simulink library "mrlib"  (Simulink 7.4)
settings: Solver=ode45  SolverMode=SingleTasking  StartTime=0.0  StopTime=10.0  RelTol=1e-3
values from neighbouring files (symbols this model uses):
  D = str2num(get(h,'string'))    [acttrcalc1.m]
  fr0 = [phidr phiqr]    [imdef0vec.m]    (also in imdef1vec.m; imdefrotflux.m = sqrt(phidr^2+phiqr^2); imdefSIvec1.m)
  fs0 = fs    [calc0.m]    (also in imdef0vec.m = [phids phiqs]; imdef1vec.m = [phids phiqs]; imdefrotflux.m = [fs0d fs0q]; imdefSIvec1.m = [phids phiqs])
  gam = 2*pi/3    (= 2.09439510239)    [IMabc2.m]    (also in IMabcf0.m; IMabcf1.m; imabcparam.m; IMabcrun0.m)
  ic = [fs0 fr0]    [imdef0vec.m]    (also in imdef1vec.m; imdef2vec.m = F; imic2.m = [phids phiqs phidr phiqr n0]'; imic3.m = [phids phiqs phidr phiqr n0]')
  Lm1 = 2/3*Lm    [IMabcf0.m]    (also in IMabcf1.m; imabcparam.m = 0.0564666666667; IMabcrun0.m = 0.0564666666667; IMabcrun1.m = 0.0564666666667)
  Lr = Lrl+Lm    (= 4.6)    [IMabc2.m]    (also in IMabcf0.m = Lrl+Lm1; IMabcf1.m = Lrl+Lm1; imabcparam.m = 0.0589666666667; IMcur0.m)
  Lrr = [Lr   -Lm/2 -Lm/2    [IMabc2.m]    (also in IMabcf0.m = [Lr   -Lm1/2 -Lm1/2; IMabcf1.m = [Lr   -Lm1/2 -Lm1/2)
  Ls = Lsl+Lm    (= 4.6)    [IMabc2.m]    (also in IMabcf0.m = Lsl+Lm1; IMabcf1.m = Lsl+Lm1; imabcparam.m = 0.0589666666667; IMcur0.m)
  Lss = [Ls   -Lm/2 -Lm/2    [IMabc2.m]    (also in IMabcf0.m = [Ls   -Lm1/2 -Lm1/2; IMabcf1.m = [Ls   -Lm1/2 -Lm1/2)
  p = cos(beta-alpha)    [abcRwdg.m]    (also in alternator.m = 0:pi/20:2*pi; altwdgs.m = 0:pi/20:2*pi; brushlessdcB.m = 0:pi/100:2*pi; brushlessdcnew.m = 0:pi/100:2*pi)
  R = str2num(get(h,'string'))    [acttrcalc1.m]    (also in IMabc2.m = diag([Rs Rs Rs Rr Rr Rr]); IMabcf0.m = diag([Rs Rs Rs Rr Rr Rr]); IMabcf1.m = diag([Rs Rs Rs Rr Rr Rr]); IMcurf0.m = diag([Rs Rs Rr Rr]))
  Ra = .95    (= 0.95)    [altwdgs.m]    (also in Ccurverun.m = 0.018)
  Rr = input('Rotor resistance)[default = 2] =')    [Actac.m]    (also in im1phase.m = 0.3; im3d.m = eval(get(hRr,'String')); IMabc2.m = 0.02; imabcparam.m = 0.408)
  Rs = eval(get(hRs,'String'))    [im3d.m]    (also in IMabc2.m = 0.01; imabcparam.m = 0.531; IMabcrun0.m = 0.531; IMabcrun1.m = 0.531)
  Vm = Vll*sqrt(2/3)    [imabcparam.m]
  wo = 2*pi*freq0    [calc0.m]    (also in IMabc2.m = 376.991118431; imabcparam.m = 376.991118431; IMabcrun0.m = 376.991118431; IMabcrun1.m = 376.991118431)
undefined symbols (not defined in the file or in its folder): fa0, fk0, ifo, L_1, Laf, Lakd, Lakq, phif0, Rf, Rkd, Rkq, Row, vector
libraries: simulink x4

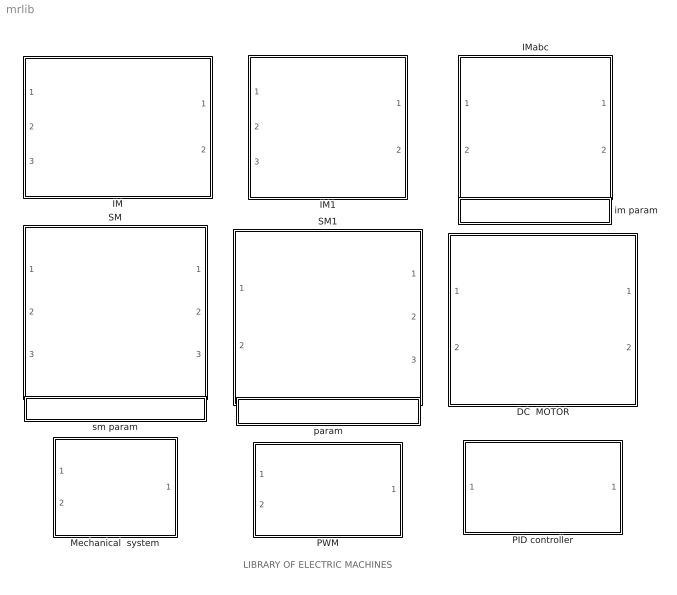
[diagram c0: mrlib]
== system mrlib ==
  note: LIBRARY OF ELECTRIC MACHINES
  DC  MOTOR : Subsystem  mask{Ra=2.0, La=5.2e-3, J=1.5e-4, Bm=1e-3, K=0.1}
      mask prompts: Ra "Armature resistance [ohm]"; La "Armature inductance [H]"; J "Moment of inertia [Kg.m^2]"; Bm "Frictional torque cefficient"; K "Electromechanical coupling coefficient [N.m/A]"
  IM : Subsystem  mask{Rs=0.02, Rr=0.01, Lsl=0.1, Lrl=0.1, Lm=5, wo=2*pi*60}
      mask prompts: Rs "Stator resistance [pu]"; Rr "Rotor resistance [pu]"; Lsl "Stator leakage inductance [pu]"; Lrl "Rotor leakage inductance [pu]"; Lm "Magnetizing inductance [pu]"; wo "Base frequency [rad/s]"
      mask help: Induction motor state space model in arbitrary reference frame. Parameters are expressed in per unit.
  IM1 : Subsystem  mask{Rs=0.5, Rr=0.5, Lsl=3e-3, Lrl=3e-3, Lm=100e-3, p=4, wo=2*pi*60}
      mask prompts: Rs "Stator resistance [Ohm]"; Rr "Rotor resistance [Ohm]"; Lsl "Stator leakage inductance [H]"; Lrl "Rotor leakage inductance [H]"; Lm "Magnetizing inductance [H]"; p "Number of poles"; wo "Base frequency [rad/s]"
  IMabc : Subsystem
  Mechanical  system : Subsystem  mask{H=0.3, B1=1e-5, B2=0, a=2}
      mask prompts: H "Inertia constant [s]"; B1 "Viscous damping coefficient"; B2 "Fan load factor"; a "Fan load exponent"
  PID controller : Subsystem  mask{Kp=1, Ki=10, Kd=0.1, sat=inf}
      mask prompts: Kp "Proportional gain (Kp)"; Ki "Integral gain (Ki)"; Kd "Derivative gain (Kd)"; sat "Saturation limit [pu]"
      mask help: Proportional-Integral Speed Controller
  PWM : Subsystem
  SM : Subsystem
  SM1 : Subsystem
  im param : Subsystem
  param : Subsystem
  sm param : Subsystem

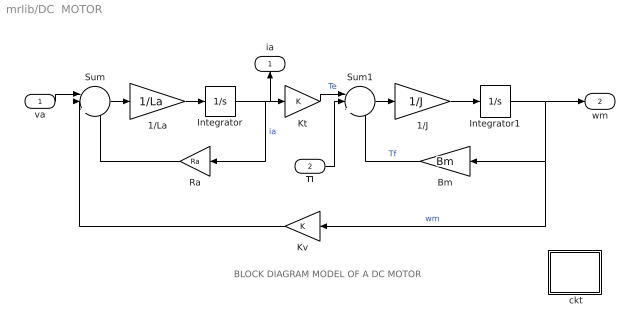
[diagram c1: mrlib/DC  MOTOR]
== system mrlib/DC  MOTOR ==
  note: BLOCK DIAGRAM MODEL OF A DC MOTOR
  va : Inport  OutDataType=sfix(16)  OutScaling=2^0
  Tl : Inport  Port=2  OutDataType=sfix(16)  OutScaling=2^0
  " ckt" : Subsystem
  1/J : Gain  Gain=1/J  ParameterDataType=sfix(16)  ParameterScaling=2^0  OutDataType=sfix(16)  OutScaling=2^0
  1/La : Gain  Gain=1/La  ParameterDataType=sfix(16)  ParameterScaling=2^0  OutDataType=sfix(16)  OutScaling=2^0
  Bm : Gain  Gain=Bm  ParameterDataType=sfix(16)  ParameterScaling=2^0  OutDataType=sfix(16)  OutScaling=2^0
  Integrator : Integrator
  Integrator1 : Integrator
  Kt : Gain  Gain=K  ParameterDataType=sfix(16)  ParameterScaling=2^0  OutDataType=sfix(16)  OutScaling=2^0
  Kv : Gain  Gain=K  ParameterDataType=sfix(16)  ParameterScaling=2^0  OutDataType=sfix(16)  OutScaling=2^0
  Ra : Gain  Gain=Ra  ParameterDataType=sfix(16)  ParameterScaling=2^0  OutDataType=sfix(16)  OutScaling=2^0
  Sum : Sum  Inputs=||+--  OutDataType=sfix(16)  OutScaling=2^0
  Sum1 : Sum  Inputs=||+--  OutDataType=sfix(16)  OutScaling=2^0
  ia : Outport
  wm : Outport  Port=2
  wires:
  Kv/1 -> Sum/2
  Ra/1 -> Sum/3
  Kt/1 -> Sum1/1  "Te"
  Bm/1 -> Sum1/3  "Tf"
  Sum/1 -> 1/La/1
  1/La/1 -> Integrator/1
  Integrator/1 -> Ra/1, Kt/1, ia/1  "ia"
  Sum1/1 -> 1/J/1
  1/J/1 -> Integrator1/1
  va/1 -> Sum/1
  Tl/1 -> Sum1/2
  Integrator1/1 -> Bm/1, Kv/1, wm/1  "wm"

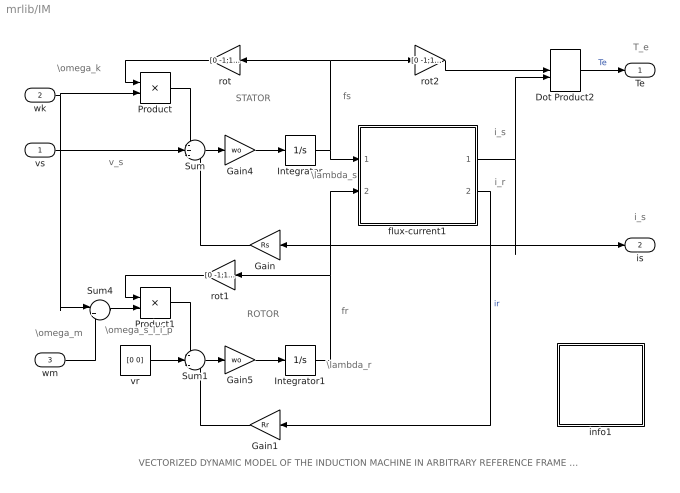
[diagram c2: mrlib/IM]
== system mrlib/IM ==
  note: VECTORIZED DYNAMIC MODEL OF THE INDUCTION MACHINE IN ARBITRARY REFERENCE FRAME (per unit formulation)
  note: fr
  note: fs
  note: STATOR
  note: ROTOR
  note: \omega_s_l_i_p
  note: T_e
  note: i_s
  note: i_s
  note: i_r
  note: \omega_m
  note: \lambda_s
  note: \lambda_r
  note: v_s
  note: \omega_k
  vs : Inport  OutDataType=sfix(16)  OutScaling=2^0
  wk : Inport  Port=2  OutDataType=sfix(16)  OutScaling=2^0
  wm : Inport  Port=3  OutDataType=sfix(16)  OutScaling=2^0
  Dot Product2 : DotProduct  OutDataType=fixdt(1, 16)  OutScaling=2^-10
  Gain : Gain  Gain=Rs  ParameterDataType=sfix(16)  ParameterScaling=2^0  OutDataType=sfix(16)  OutScaling=2^0
  Gain1 : Gain  Gain=Rr  ParameterDataType=sfix(16)  ParameterScaling=2^0  OutDataType=sfix(16)  OutScaling=2^0
  Gain4 : Gain  Gain=wo  ParameterDataType=sfix(16)  ParameterScaling=2^0  OutDataType=sfix(16)  OutScaling=2^0
  Gain5 : Gain  Gain=wo  ParameterDataType=sfix(16)  ParameterScaling=2^0  OutDataType=sfix(16)  OutScaling=2^0
  Integrator : Integrator  InitialCondition=[ic(1) ic(2)]
  Integrator1 : Integrator  InitialCondition=[ic(3) ic(4)]
  Product : Product  OutDataType=sfix(16)  OutScaling=2^0
  Product1 : Product  OutDataType=sfix(16)  OutScaling=2^0
  Sum : Sum  Inputs=-+-  OutDataType=sfix(16)  OutScaling=2^0
  Sum1 : Sum  Inputs=-+-  OutDataType=sfix(16)  OutScaling=2^0
  Sum4 : Sum  Inputs=|+-  OutDataType=sfix(16)  OutScaling=2^0
  flux-current1 : Subsystem
  info1 : Subsystem
  rot : Gain  Gain=[0 -1;1 0]  Multiplication=Matrix(K*u)  ParameterDataType=sfix(16)  ParameterScaling=2^0  OutDataType=sfix(16)  OutScaling=2^0
  rot1 : Gain  Gain=[0 -1;1 0]  Multiplication=Matrix(K*u)  ParameterDataType=sfix(16)  ParameterScaling=2^0  OutDataType=sfix(16)  OutScaling=2^0
  rot2 : Gain  Gain=[0 -1;1 0]  Multiplication=Matrix(K*u)  ParameterDataType=sfix(16)  ParameterScaling=2^0  OutDataType=sfix(16)  OutScaling=2^0
  vr : Constant  Value=[0 0]  OutDataType=sfix(16)  OutScaling=2^0
  Te : Outport
  is : Outport  Port=2
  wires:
  wm/1 -> Sum4/2
  wk/1 -> Sum4/1, Product/2
  vs/1 -> Sum/2
  Dot Product2/1 -> Te/1  "Te"
  flux-current1/1(is) -> Dot Product2/2, is/1, Gain/1
  Gain5/1 -> Integrator1/1
  Sum1/1 -> Gain5/1
  Gain4/1 -> Integrator/1
  Sum/1 -> Gain4/1
  Sum4/1 -> Product1/2
  rot2/1 -> Dot Product2/1
  rot/1 -> Product/1
  Product/1 -> Sum/1
  rot1/1 -> Product1/1
  Product1/1 -> Sum1/1
  Integrator1/1 -> flux-current1/2(fr), rot1/1
  Integrator/1 -> rot2/1, rot/1, flux-current1/1(fs)
  flux-current1/2(ir) -> Gain1/1  "ir"
  Gain1/1 -> Sum1/3
  vr/1 -> Sum1/2
  Gain/1 -> Sum/3

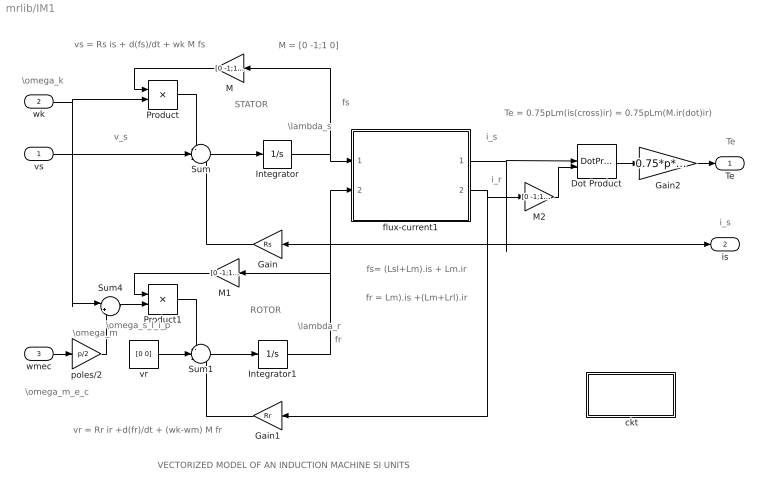
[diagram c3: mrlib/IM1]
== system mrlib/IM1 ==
  note: ROTOR
  note: STATOR
  note: fs
  note: VECTORIZED MODEL OF AN INDUCTION MACHINE SI UNITS
  note: vs = Rs is + d(fs)/dt + wk M fs
  note: vr = Rr ir +d(fr)/dt + (wk-wm) M fr
  note: fs= (Lsl+Lm).is + Lm.ir
  note: fr = Lm).is +(Lm+Lrl).ir
  note: Te = 0.75pLm(is(cross)ir) = 0.75pLm(M.ir(dot)ir)
  note: M = [0 -1;1 0]
  note: fr
  note: Te
  note: \lambda_s
  note: \lambda_r
  note: i_s
  note: i_s
  note: i_r
  note: \omega_m
  note: \omega_m_e_c
  note: \omega_k
  note: v_s
  note: \omega_s_l_i_p
  vs : Inport  OutDataType=sfix(16)  OutScaling=2^0
  wk : Inport  Port=2  OutDataType=sfix(16)  OutScaling=2^0
  wmec : Inport  Port=3  OutDataType=sfix(16)  OutScaling=2^0
  " ckt" : Subsystem
  Dot Product : DotProduct  OutDataType=fixdt(1, 16)  OutScaling=2^-10
  Gain : Gain  Gain=Rs  ParameterDataType=sfix(16)  ParameterScaling=2^0  OutDataType=sfix(16)  OutScaling=2^0
  Gain1 : Gain  Gain=Rr  ParameterDataType=sfix(16)  ParameterScaling=2^0  OutDataType=sfix(16)  OutScaling=2^0
  Gain2 : Gain  Gain=0.75*p*Lm  ParameterDataType=sfix(16)  ParameterScaling=2^0  OutDataType=sfix(16)  OutScaling=2^0
  Integrator : Integrator  InitialCondition=fs0
  Integrator1 : Integrator  InitialCondition=fr0
  M : Gain  Gain=[0 -1;1 0]  Multiplication=Matrix(K*u)  ParameterDataType=sfix(16)  ParameterScaling=2^0  OutDataType=sfix(16)  OutScaling=2^0
  M1 : Gain  Gain=[0 -1;1 0]  Multiplication=Matrix(K*u)  ParameterDataType=sfix(16)  ParameterScaling=2^0  OutDataType=sfix(16)  OutScaling=2^0
  M2 : Gain  Gain=[0 -1;1 0]  Multiplication=Matrix(K*u)  ParameterDataType=sfix(16)  ParameterScaling=2^0  OutDataType=sfix(16)  OutScaling=2^0
  Product : Product  OutDataType=sfix(16)  OutScaling=2^0
  Product1 : Product  OutDataType=sfix(16)  OutScaling=2^0
  Sum : Sum  Inputs=-+-  OutDataType=sfix(16)  OutScaling=2^0
  Sum1 : Sum  Inputs=-+-  OutDataType=sfix(16)  OutScaling=2^0
  Sum4 : Sum  Inputs=|+-  OutDataType=sfix(16)  OutScaling=2^0
  flux-current1 : Subsystem
  poles/2 : Gain  Gain=p/2  ParameterDataType=sfix(16)  ParameterScaling=2^0  OutDataType=sfix(16)  OutScaling=2^0
  vr : Constant  Value=[0 0]  OutDataType=sfix(16)  OutScaling=2^0
  Te : Outport
  is : Outport  Port=2
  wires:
  Gain/1 -> Sum/3
  vr/1 -> Sum1/2
  Gain1/1 -> Sum1/3
  Integrator/1 -> M/1, flux-current1/1(fs)
  Integrator1/1 -> flux-current1/2(fr), M1/1
  Product1/1 -> Sum1/1
  M1/1 -> Product1/1
  Product/1 -> Sum/1
  M/1 -> Product/1
  Sum4/1 -> Product1/2
  vs/1 -> Sum/2
  wk/1 -> Product/2, Sum4/1
  Sum1/1 -> Integrator1/1
  Sum/1 -> Integrator/1
  flux-current1/1(is) -> Gain/1, is/1, Dot Product/1
  Dot Product/1 -> Gain2/1
  Gain2/1 -> Te/1
  wmec/1 -> poles/2/1
  poles/2/1 -> Sum4/2
  M2/1 -> Dot Product/2
  flux-current1/2(ir) -> M2/1, Gain1/1

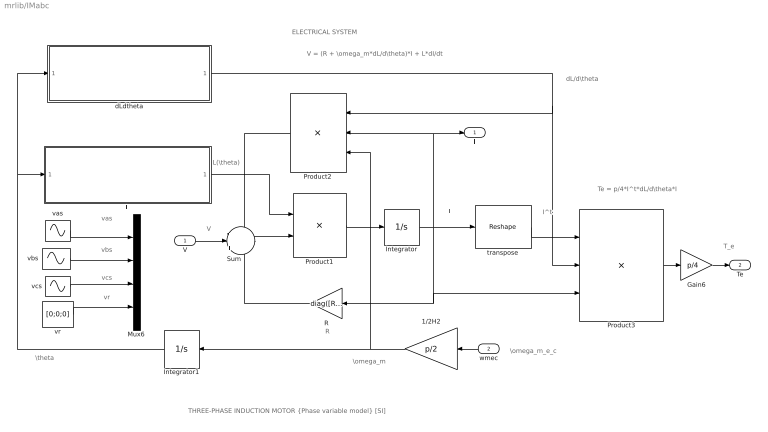
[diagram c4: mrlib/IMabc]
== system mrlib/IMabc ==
  note: I
  note: I^t
  note: ELECTRICAL SYSTEM
  note: V
  note: \omega_m
  note: \theta
  note: T_e
  note: dL/d\theta
  note: R
  note: V = (R + \omega_m*dL/d\theta)*I + L*dI/dt
  note: Te = p/4*I^t*dL/d\theta*I
  note: L(\theta)
  note: \omega_m_e_c
  note: THREE-PHASE INDUCTION MOTOR {Phase variable model} [SI]
  note: vas
  note: vbs
  note: vcs
  note: vr
  V : Inport  OutDataType=sfix(16)  OutScaling=2^0
  wmec : Inport  Port=2  OutDataType=sfix(16)  OutScaling=2^0
  1/2H2 : Gain  Gain=p/2  ParameterDataType=sfix(16)  ParameterScaling=2^0  OutDataType=sfix(16)  OutScaling=2^0
  Gain6 : Gain  Gain=p/4  ParameterDataType=sfix(16)  ParameterScaling=2^0  OutDataType=sfix(16)  OutScaling=2^0
  Integrator : Integrator  InitialCondition=[0 ;0 ;0; 0 ;0 ;0]
  Integrator1 : Integrator
  L : Subsystem
  Mux6 : Mux
  Product1 : Product  Inputs=/*  Multiplication=Matrix(*)  OutDataType=sfix(16)  OutScaling=2^0
  Product2 : Product  Inputs=***  Multiplication=Matrix(*)  OutDataType=sfix(16)  OutScaling=2^0
  Product3 : Product  Inputs=3  Multiplication=Matrix(*)  OutDataType=sfix(16)  OutScaling=2^0
  R : Gain  Gain=diag([Rs Rs Rs Rr Rr Rr])  Multiplication=Matrix(K*u)  ParameterDataType=sfix(16)  ParameterScaling=2^0  OutDataType=sfix(16)  OutScaling=2^0
  Sum : Sum  Inputs=-|+|-  OutDataType=sfix(16)  OutScaling=2^0
  dLdtheta : Subsystem
  transpose : Reshape  OutputDimensionality=Row vector (2-D)  OutputDimensions=[1,6]
  vas : Sin  Amplitude=Vm  Bias=0  Frequency=wo  Phase=pi/2  Samples=10  SampleTime=0
  vbs : Sin  Amplitude=Vm  Bias=0  Frequency=wo  Phase=pi/2-gam  Samples=10  SampleTime=0
  vcs : Sin  Amplitude=Vm  Bias=0  Frequency=wo  Phase=pi/2+gam  Samples=10  SampleTime=0
  vr : Constant  Value=[0;0;0]  VectorParams1D=off  OutDataType=sfix(16)  OutScaling=2^0
  I : Outport
  Te : Outport  Port=2
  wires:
  Product1/1 -> Integrator/1
  Integrator/1 -> Product3/3, R/1, transpose/1, Product2/2, I/1
  Sum/1 -> Product1/2
  R/1 -> Sum/3
  transpose/1 -> Product3/1
  Product2/1 -> Sum/1
  dLdtheta/1(dLdtheta) -> Product3/2, Product2/1
  Product3/1 -> Gain6/1
  1/2H2/1 -> Integrator1/1, Product2/3
  Integrator1/1 -> dLdtheta/1(theta1), L/1(theta)
  L/1(L) -> Product1/1
  V/1 -> Sum/2
  Gain6/1 -> Te/1
  wmec/1 -> 1/2H2/1
  vr/1 -> Mux6/4
  vcs/1 -> Mux6/3
  vbs/1 -> Mux6/2
  vas/1 -> Mux6/1
  Mux6/1 -> ?

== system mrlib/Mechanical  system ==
  note: fan-type load
  Tl : Inport  OutDataType=sfix(16)  OutScaling=2^0
  Te : Inport  Port=2  OutDataType=sfix(16)  OutScaling=2^0
  1/2H : Gain  Gain=1/(2*H)  ParameterDataType=sfix(16)  ParameterScaling=2^0  OutDataType=sfix(16)  OutScaling=2^0
  Bm : Gain  Gain=B1  ParameterDataType=sfix(16)  ParameterScaling=2^0  OutDataType=sfix(16)  OutScaling=2^0
  Integrator : Integrator  InitialCondition=.82
  Sum : Sum  Inputs=-+-  OutDataType=sfix(16)  OutScaling=2^0
  Sum1 : Sum  Inputs=|++  OutDataType=sfix(16)  OutScaling=2^0
  Tm : Fcn  Expr=B2*abs(u)^a
  wm : Outport
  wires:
  Tl/1 -> Sum/1
  Te/1 -> Sum/2
  Integrator/1 -> wm/1, Bm/1, Tm/1
  Sum/1 -> 1/2H/1
  1/2H/1 -> Integrator/1
  Bm/1 -> Sum1/1
  Sum1/1 -> Sum/3
  Tm/1 -> Sum1/2

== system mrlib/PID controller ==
  note: antiwindup by clamping integrator
  note: limiter
  error : Inport  OutDataType=sfix(16)  OutScaling=2^0
  Derivative : Derivative
  Gain : Gain  Gain=Ki  ParameterDataType=sfix(16)  ParameterScaling=2^0  OutDataType=sfix(16)  OutScaling=2^0
  Gain1 : Gain  Gain=Kp  ParameterDataType=sfix(16)  ParameterScaling=2^0  OutDataType=sfix(16)  OutScaling=2^0
  Gain2 : Gain  Gain=Kd  ParameterDataType=sfix(16)  ParameterScaling=2^0  OutDataType=sfix(16)  OutScaling=2^0
  Integrator : Integrator  LimitOutput=on  UpperSaturationLimit=sat  LowerSaturationLimit=-sat
  Saturation : Saturate  UpperLimit=sat  LowerLimit=-sat
  Sum : Sum  Inputs=+++  OutDataType=sfix(16)  OutScaling=2^0
  control : Outport  InitialOutput=0
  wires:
  Gain1/1 -> Sum/1
  Gain/1 -> Integrator/1
  error/1 -> Gain/1, Gain1/1, Gain2/1
  Sum/1 -> Saturation/1
  Saturation/1 -> control/1
  Integrator/1 -> Sum/2
  Gain2/1 -> Derivative/1
  Derivative/1 -> Sum/3

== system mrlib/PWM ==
  control : Inport  OutDataType=sfix(16)  OutScaling=2^0
  frequency : Inport  Port=2  OutDataType=sfix(16)  OutScaling=2^0
  Clock : Clock
  Mux : Mux  Inputs=2
  Sum2 : Sum  Inputs=|+-  OutDataType=sfix(16)  OutScaling=2^0
  saw : Fcn  Expr=1/pi*atan(tan((2*pi*u(1)*u(2)-pi)/2))+0.5
  step : Relay  OutDataType=sfix(16)  OutScaling=2^0
  Output : Outport
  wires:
  Clock/1 -> Mux/2
  Mux/1 -> saw/1
  control/1 -> Sum2/1
  frequency/1 -> Mux/1
  saw/1 -> Sum2/2
  step/1 -> Output/1
  Sum2/1 -> step/1

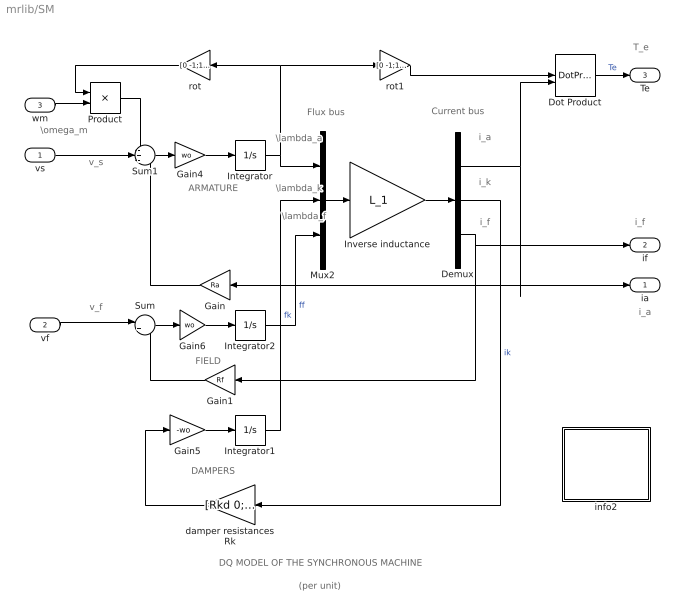
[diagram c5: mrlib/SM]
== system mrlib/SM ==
  note: DAMPERS
  note: ARMATURE
  note: i_f
  note: FIELD
  note: DQ MODEL OF THE SYNCHRONOUS MACHINE
  note: Flux bus
  note: Current bus
  note: (per unit)
  note: v_s
  note: T_e
  note: \lambda_a
  note: \lambda_k
  note: \lambda_f
  note: \omega_m
  note: v_f
  note: i_k
  note: i_a
  note: i_a
  note: i_f
  vs : Inport  OutDataType=sfix(16)  OutScaling=2^0
  vf : Inport  Port=2  OutDataType=sfix(16)  OutScaling=2^0
  wm : Inport  Port=3  OutDataType=sfix(16)  OutScaling=2^0
  Demux : Demux  Outputs=3
  Dot Product : DotProduct  OutDataType=fixdt(1, 16)  OutScaling=2^-10
  Gain : Gain  Gain=Ra  ParameterDataType=sfix(16)  ParameterScaling=2^0  OutDataType=sfix(16)  OutScaling=2^0
  Gain1 : Gain  Gain=Rf  ParameterDataType=sfix(16)  ParameterScaling=2^0  OutDataType=sfix(16)  OutScaling=2^0
  Gain4 : Gain  Gain=wo  ParameterDataType=sfix(16)  ParameterScaling=2^0  OutDataType=sfix(16)  OutScaling=2^0
  Gain5 : Gain  Gain=-wo  ParameterDataType=sfix(16)  ParameterScaling=2^0  OutDataType=sfix(16)  OutScaling=2^0
  Gain6 : Gain  Gain=wo  ParameterDataType=sfix(16)  ParameterScaling=2^0  OutDataType=sfix(16)  OutScaling=2^0
  Integrator : Integrator  InitialCondition=fa0
  Integrator1 : Integrator  InitialCondition=fk0
  Integrator2 : Integrator  InitialCondition=phif0
  Inverse inductance : Gain  Gain=L_1  Multiplication=Matrix(K*u)  ParameterDataType=sfix(16)  ParameterScaling=2^0  OutDataType=sfix(16)  OutScaling=2^0
  Mux2 : Mux  Inputs=3
  Product : Product  OutDataType=sfix(16)  OutScaling=2^0
  Sum : Sum  Inputs=|+-  OutDataType=sfix(16)  OutScaling=2^0
  Sum1 : Sum  Inputs=-+-  OutDataType=sfix(16)  OutScaling=2^0
  damper resistances Rk : Gain  Gain=[Rkd 0;0 Rkq]  Multiplication=Matrix(K*u)  ParameterDataType=sfix(16)  ParameterScaling=2^0  OutDataType=sfix(16)  OutScaling=2^0
  info2 : Subsystem
  rot : Gain  Gain=[0 -1;1 0]  Multiplication=Matrix(K*u)  ParameterDataType=sfix(16)  ParameterScaling=2^0  OutDataType=sfix(16)  OutScaling=2^0
  rot1 : Gain  Gain=[0 -1;1 0]  Multiplication=Matrix(K*u)  ParameterDataType=sfix(16)  ParameterScaling=2^0  OutDataType=sfix(16)  OutScaling=2^0
  ia : Outport
  if : Outport  Port=2
  Te : Outport  Port=3
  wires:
  Product/1 -> Sum1/1
  rot/1 -> Product/1
  Gain5/1 -> Integrator1/1
  damper resistances Rk/1 -> Gain5/1
  Integrator/1 -> Mux2/1, rot/1, rot1/1
  Sum1/1 -> Gain4/1
  Gain4/1 -> Integrator/1
  vs/1 -> Sum1/2
  Gain/1 -> Sum1/3
  Gain6/1 -> Integrator2/1
  Sum/1 -> Gain6/1
  vf/1 -> Sum/1
  Gain1/1 -> Sum/2
  rot1/1 -> Dot Product/1
  Demux/1 -> Gain/1, ia/1, Dot Product/2
  Dot Product/1 -> Te/1  "Te"
  Mux2/1 -> Inverse inductance/1
  Inverse inductance/1 -> Demux/1
  Integrator1/1 -> Mux2/2  "fk"
  Integrator2/1 -> Mux2/3  "ff"
  Demux/2 -> damper resistances Rk/1  "ik"
  Demux/3 -> if/1, Gain1/1
  wm/1 -> Product/2

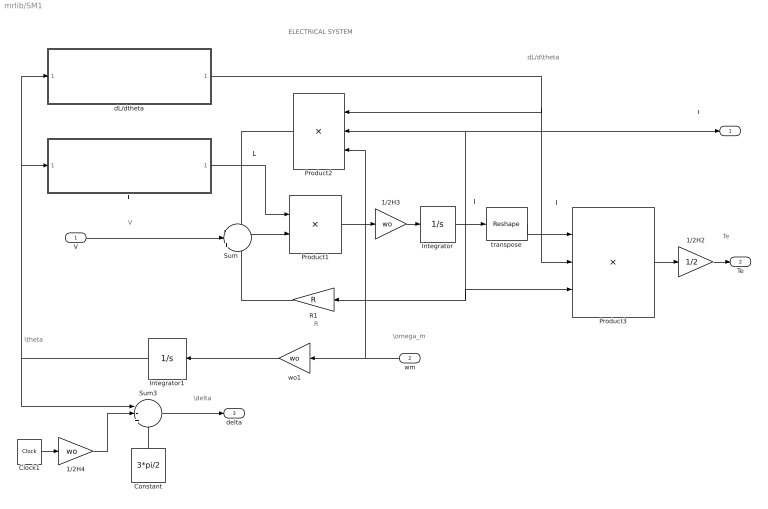
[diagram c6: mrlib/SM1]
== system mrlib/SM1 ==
  note: \theta
  note: dL/d\theta
  note: L
  note: V
  note: ELECTRICAL SYSTEM
  note: I'
  note: I
  note: Te
  note: I
  note: \omega_m
  note: R
  note: \delta
  V : Inport  OutDataType=sfix(16)  OutScaling=2^0
  wm : Inport  Port=2  OutDataType=sfix(16)  OutScaling=2^0
  1/2H2 : Gain  Gain=1/2  ParameterDataType=sfix(16)  ParameterScaling=2^0  OutDataType=sfix(16)  OutScaling=2^0
  1/2H3 : Gain  Gain=wo  ParameterDataType=sfix(16)  ParameterScaling=2^0  OutDataType=sfix(16)  OutScaling=2^0
  1/2H4 : Gain  Gain=wo  ParameterDataType=sfix(16)  ParameterScaling=2^0  OutDataType=sfix(16)  OutScaling=2^0
  Clock1 : Clock
  Constant : Constant  Value=3*pi/2  OutDataType=sfix(16)  OutScaling=2^0
  Integrator : Integrator  InitialCondition="[-0.0133    0.0414   -0.0281    ifo   0.0000    0.0000  ]'"  ZeroCross=off
  Integrator1 : Integrator  InitialCondition=4.7323
  L : Subsystem
  Product1 : Product  Inputs=/*  Multiplication=Matrix(*)  OutDataType=sfix(16)  OutScaling=2^0
  Product2 : Product  Inputs=***  Multiplication=Matrix(*)  OutDataType=sfix(16)  OutScaling=2^0
  Product3 : Product  Inputs=3  Multiplication=Matrix(*)  OutDataType=sfix(16)  OutScaling=2^0
  R1 : Gain  Gain=R  Multiplication=Matrix(K*u)  ParameterDataType=sfix(16)  ParameterScaling=2^0  OutDataType=sfix(16)  OutScaling=2^0
  Sum : Sum  Inputs=-|+|-  OutDataType=sfix(16)  OutScaling=2^0
  Sum3 : Sum  Inputs=|-++  OutDataType=sfix(16)  OutScaling=2^0
  dL/dtheta : Subsystem
  transpose : Reshape  OutputDimensionality=Row vector (2-D)  OutputDimensions=[1,6]
  wo1 : Gain  Gain=wo  ParameterDataType=sfix(16)  ParameterScaling=2^0  OutDataType=sfix(16)  OutScaling=2^0
  I : Outport
  Te : Outport  Port=2
  delta : Outport  Port=3
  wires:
  wo1/1 -> Integrator1/1
  R1/1 -> Sum/3
  1/2H3/1 -> Integrator/1
  Integrator/1 -> transpose/1, Product2/2, I/1, R1/1, Product3/3
  L/1(L) -> Product1/1
  Integrator1/1 -> dL/dtheta/1(theta1), L/1(theta), Sum3/1
  Product3/1 -> 1/2H2/1
  dL/dtheta/1(dLdtheta) -> Product2/1, Product3/2
  Product2/1 -> Sum/1
  transpose/1 -> Product3/1
  Sum/1 -> Product1/2
  Product1/1 -> 1/2H3/1
  wm/1 -> Product2/3, wo1/1
  V/1 -> Sum/2
  1/2H2/1 -> Te/1
  Clock1/1 -> 1/2H4/1
  1/2H4/1 -> Sum3/2
  Constant/1 -> Sum3/3
  Sum3/1 -> delta/1

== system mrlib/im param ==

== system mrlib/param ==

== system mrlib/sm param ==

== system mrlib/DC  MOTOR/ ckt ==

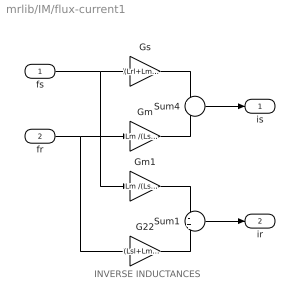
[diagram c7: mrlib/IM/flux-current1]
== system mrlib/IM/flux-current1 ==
  note: INVERSE INDUCTANCES
  fs : Inport  OutDataType=sfix(16)  OutScaling=2^0
  fr : Inport  Port=2  OutDataType=sfix(16)  OutScaling=2^0
  G22 : Gain  Gain=(Lsl+Lm )/(Lsl*Lrl+Lsl*Lm+Lrl*Lm)  ParameterDataType=sfix(16)  ParameterScaling=2^0  OutDataType=sfix(16)  OutScaling=2^0
  Gm : Gain  Gain=Lm /(Lsl*Lrl+Lsl*Lm+Lrl*Lm)  ParameterDataType=sfix(16)  ParameterScaling=2^0  OutDataType=sfix(16)  OutScaling=2^0
  Gm1 : Gain  Gain=Lm /(Lsl*Lrl+Lsl*Lm+Lrl*Lm)  ParameterDataType=sfix(16)  ParameterScaling=2^0  OutDataType=sfix(16)  OutScaling=2^0
  Gs : Gain  Gain=(Lrl+Lm) /(Lsl*Lrl+Lsl*Lm+Lrl*Lm)  ParameterDataType=sfix(16)  ParameterScaling=2^0  OutDataType=sfix(16)  OutScaling=2^0
  Sum1 : Sum  Inputs=-+  OutDataType=sfix(16)  OutScaling=2^0
  Sum4 : Sum  Inputs=+-  OutDataType=sfix(16)  OutScaling=2^0
  is : Outport
  ir : Outport  Port=2
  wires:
  Sum1/1 -> ir/1
  G22/1 -> Sum1/2
  Gm1/1 -> Sum1/1
  Sum4/1 -> is/1
  Gm/1 -> Sum4/2
  fr/1 -> G22/1, Gm/1
  Gs/1 -> Sum4/1
  fs/1 -> Gm1/1, Gs/1

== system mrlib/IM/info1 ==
  note: This demonstration illustrates the dynamics of a synchronous generator, initially at no load, following a three-phase short circuit at the terminals.
  note: Synchronous machine transients under shortcircuit

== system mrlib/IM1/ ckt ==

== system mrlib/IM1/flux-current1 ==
  note: INVERSE INDUCTANCE
  fs : Inport  OutDataType=sfix(16)  OutScaling=2^0
  fr : Inport  Port=2  OutDataType=sfix(16)  OutScaling=2^0
  Gm : Gain  Gain=Lm /(Lsl*Lrl+Lsl*Lm+Lrl*Lm)  ParameterDataType=sfix(16)  ParameterScaling=2^0  OutDataType=sfix(16)  OutScaling=2^0
  Gm1 : Gain  Gain=Lm /(Lsl*Lrl+Lsl*Lm+Lrl*Lm)  ParameterDataType=sfix(16)  ParameterScaling=2^0  OutDataType=sfix(16)  OutScaling=2^0
  Gr : Gain  Gain=(Lsl+Lm )/(Lsl*Lrl+Lsl*Lm+Lrl*Lm)  ParameterDataType=sfix(16)  ParameterScaling=2^0  OutDataType=sfix(16)  OutScaling=2^0
  Gs : Gain  Gain=(Lrl+Lm) /(Lsl*Lrl+Lsl*Lm+Lrl*Lm)  ParameterDataType=sfix(16)  ParameterScaling=2^0  OutDataType=sfix(16)  OutScaling=2^0
  Sum1 : Sum  Inputs=-+  OutDataType=sfix(16)  OutScaling=2^0
  Sum4 : Sum  Inputs=+-  OutDataType=sfix(16)  OutScaling=2^0
  is : Outport
  ir : Outport  Port=2
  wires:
  fs/1 -> Gs/1, Gm1/1
  Gs/1 -> Sum4/1
  fr/1 -> Gm/1, Gr/1
  Gm/1 -> Sum4/2
  Sum4/1 -> is/1
  Gm1/1 -> Sum1/1
  Gr/1 -> Sum1/2
  Sum1/1 -> ir/1

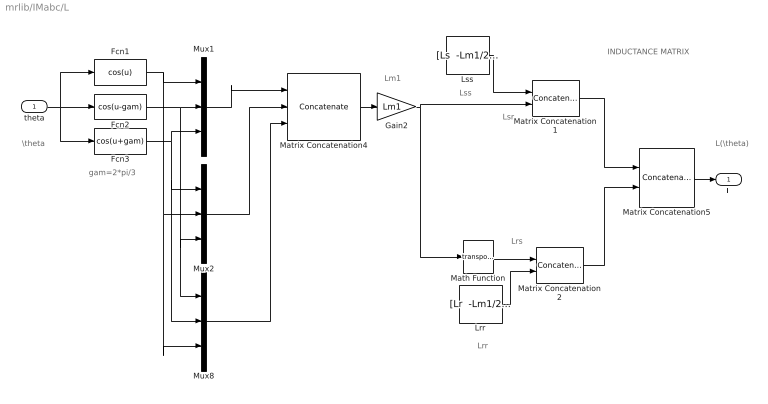
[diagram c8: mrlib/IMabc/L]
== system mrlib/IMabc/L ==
  note: INDUCTANCE MATRIX
  note: L(\theta)
  note: \theta
  note: gam=2*pi/3
  note: Lrr
  note: Lss
  note: Lsr
  note: Lrs
  note: Lm1
  theta : Inport  OutDataType=sfix(16)  OutScaling=2^0
  Fcn1 : Fcn  Expr=cos(u)
  Fcn2 : Fcn  Expr=cos(u-gam)
  Fcn3 : Fcn  Expr=cos(u+gam)
  Gain2 : Gain  Gain=Lm1  ParameterDataType=sfix(16)  ParameterScaling=2^0  OutDataType=sfix(16)  OutScaling=2^0
  Lrr : Constant  Value="[Lr  -Lm1/2  -Lm1/2; -Lm1/2  Lr -Lm1/2;-Lm1/2  -Lm1/2  Lr]"  VectorParams1D=off  OutDataType=sfix(16)  OutScaling=2^0
  Lss : Constant  Value="[Ls  -Lm1/2  -Lm1/2; -Lm1/2  Ls  -Lm1/2;-Lm1/2  -Lm1/2  Ls]"  VectorParams1D=off  OutDataType=sfix(16)  OutScaling=2^0
  Math Function : Math  Operator=transpose
  Matrix Concatenation1 : Concatenate  Mode=Multidimensional array  ConcatenateDimension=2
  Matrix Concatenation2 : Concatenate  Mode=Multidimensional array  ConcatenateDimension=2
  Matrix Concatenation4 : Concatenate  NumInputs=3  Mode=Multidimensional array  ConcatenateDimension=2
  Matrix Concatenation5 : Concatenate  Mode=Multidimensional array
  Mux1 : Mux  Inputs=3
  Mux2 : Mux  Inputs=3
  Mux8 : Mux  Inputs=3
  L : Outport
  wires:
  Matrix Concatenation5/1 -> L/1
  theta/1 -> Fcn3/1, Fcn1/1, Fcn2/1
  Math Function/1 -> Matrix Concatenation2/1
  Gain2/1 -> Matrix Concatenation1/2, Math Function/1
  Mux1/1 -> Matrix Concatenation4/1
  Matrix Concatenation4/1 -> Gain2/1
  Mux8/1 -> Matrix Concatenation4/3
  Mux2/1 -> Matrix Concatenation4/2
  Matrix Concatenation1/1 -> Matrix Concatenation5/1
  Matrix Concatenation2/1 -> Matrix Concatenation5/2
  Lss/1 -> Matrix Concatenation1/1
  Lrr/1 -> Matrix Concatenation2/2
  Fcn3/1 -> Mux1/3, Mux2/1, Mux8/2
  Fcn2/1 -> Mux1/2, Mux2/3, Mux8/1
  Fcn1/1 -> Mux8/3, Mux2/2, Mux1/1

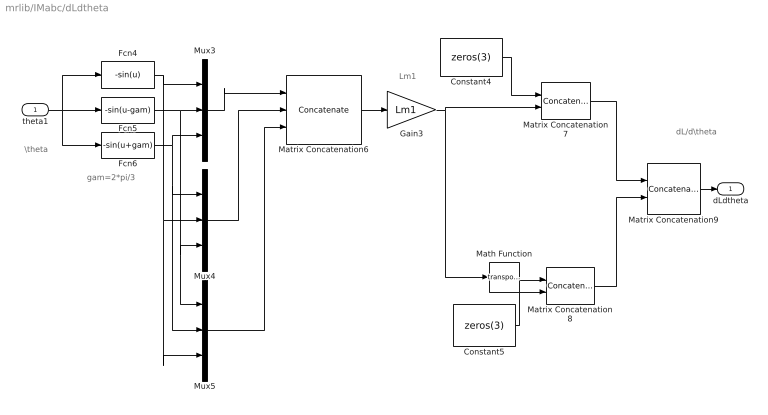
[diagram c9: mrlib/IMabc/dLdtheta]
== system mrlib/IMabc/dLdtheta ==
  note: dL/d\theta
  note: \theta
  note: gam=2*pi/3
  note: Lm1
  theta1 : Inport  OutDataType=sfix(16)  OutScaling=2^0
  Constant4 : Constant  Value=zeros(3)  VectorParams1D=off  OutDataType=sfix(16)  OutScaling=2^0
  Constant5 : Constant  Value=zeros(3)  VectorParams1D=off  OutDataType=sfix(16)  OutScaling=2^0
  Fcn4 : Fcn  Expr=-sin(u)
  Fcn5 : Fcn  Expr=-sin(u-gam)
  Fcn6 : Fcn  Expr=-sin(u+gam)
  Gain3 : Gain  Gain=Lm1  ParameterDataType=sfix(16)  ParameterScaling=2^0  OutDataType=sfix(16)  OutScaling=2^0
  Math Function : Math  Operator=transpose
  Matrix Concatenation6 : Concatenate  NumInputs=3  Mode=Multidimensional array  ConcatenateDimension=2
  Matrix Concatenation7 : Concatenate  Mode=Multidimensional array  ConcatenateDimension=2
  Matrix Concatenation8 : Concatenate  Mode=Multidimensional array  ConcatenateDimension=2
  Matrix Concatenation9 : Concatenate  Mode=Multidimensional array
  Mux3 : Mux  Inputs=3
  Mux4 : Mux  Inputs=3
  Mux5 : Mux  Inputs=3
  dLdtheta : Outport
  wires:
  Matrix Concatenation9/1 -> dLdtheta/1
  theta1/1 -> Fcn5/1, Fcn4/1, Fcn6/1
  Gain3/1 -> Matrix Concatenation7/2, Math Function/1
  Mux4/1 -> Matrix Concatenation6/2
  Mux3/1 -> Matrix Concatenation6/1
  Matrix Concatenation6/1 -> Gain3/1
  Mux5/1 -> Matrix Concatenation6/3
  Matrix Concatenation7/1 -> Matrix Concatenation9/1
  Matrix Concatenation8/1 -> Matrix Concatenation9/2
  Constant4/1 -> Matrix Concatenation7/1
  Constant5/1 -> Matrix Concatenation8/2
  Fcn6/1 -> Mux3/3, Mux4/1, Mux5/2
  Fcn5/1 -> Mux3/2, Mux4/3, Mux5/1
  Fcn4/1 -> Mux3/1, Mux4/2, Mux5/3
  Math Function/1 -> Matrix Concatenation8/1

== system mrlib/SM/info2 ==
  note: Synchronous machine transients under shortcircuit
  note: This demonstration illustrates the dynamics of a synchronous generator, initially at no load, following a three-phase short circuit at the terminals.

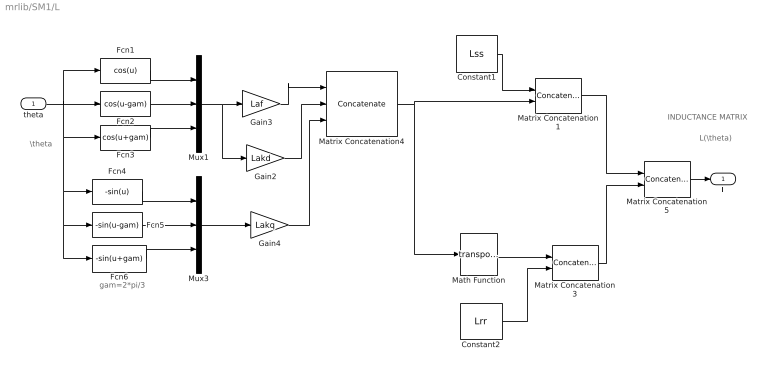
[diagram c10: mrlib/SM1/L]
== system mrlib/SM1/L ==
  note: INDUCTANCE MATRIX
  note: gam=2*pi/3
  note: \theta
  note: L(\theta)
  theta : Inport  OutDataType=sfix(16)  OutScaling=2^0
  Constant1 : Constant  Value=Lss  VectorParams1D=off  OutDataType=sfix(16)  OutScaling=2^0
  Constant2 : Constant  Value=Lrr  VectorParams1D=off  OutDataType=sfix(16)  OutScaling=2^0
  Fcn1 : Fcn  Expr=cos(u)
  Fcn2 : Fcn  Expr=cos(u-gam)
  Fcn3 : Fcn  Expr=cos(u+gam)
  Fcn4 : Fcn  Expr=-sin(u)
  Fcn5 : Fcn  Expr=-sin(u-gam)
  Fcn6 : Fcn  Expr=-sin(u+gam)
  Gain2 : Gain  Gain=Lakd  ParameterDataType=sfix(16)  ParameterScaling=2^0  OutDataType=sfix(16)  OutScaling=2^0
  Gain3 : Gain  Gain=Laf  ParameterDataType=sfix(16)  ParameterScaling=2^0  OutDataType=sfix(16)  OutScaling=2^0
  Gain4 : Gain  Gain=Lakq  ParameterDataType=sfix(16)  ParameterScaling=2^0  OutDataType=sfix(16)  OutScaling=2^0
  Math Function : Math  Operator=transpose
  Matrix Concatenation1 : Concatenate  Mode=Multidimensional array  ConcatenateDimension=2
  Matrix Concatenation3 : Concatenate  Mode=Multidimensional array  ConcatenateDimension=2
  Matrix Concatenation4 : Concatenate  NumInputs=3  Mode=Multidimensional array  ConcatenateDimension=2
  Matrix Concatenation5 : Concatenate  Mode=Multidimensional array
  Mux1 : Mux  Inputs=3
  Mux3 : Mux  Inputs=3
  L : Outport
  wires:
  Matrix Concatenation5/1 -> L/1
  Matrix Concatenation4/1 -> Matrix Concatenation1/2, Math Function/1
  Mux1/1 -> Gain3/1, Gain2/1
  Matrix Concatenation1/1 -> Matrix Concatenation5/1
  Constant1/1 -> Matrix Concatenation1/1
  Fcn3/1 -> Mux1/3
  Fcn2/1 -> Mux1/2
  Fcn1/1 -> Mux1/1
  theta/1 -> Fcn2/1, Fcn1/1, Fcn3/1, Fcn6/1, Fcn5/1, Fcn4/1
  Gain3/1 -> Matrix Concatenation4/1
  Gain2/1 -> Matrix Concatenation4/2
  Fcn5/1 -> Mux3/2
  Fcn4/1 -> Mux3/1
  Fcn6/1 -> Mux3/3
  Mux3/1 -> Gain4/1
  Gain4/1 -> Matrix Concatenation4/3
  Math Function/1 -> Matrix Concatenation3/1
  Constant2/1 -> Matrix Concatenation3/2
  Matrix Concatenation3/1 -> Matrix Concatenation5/2

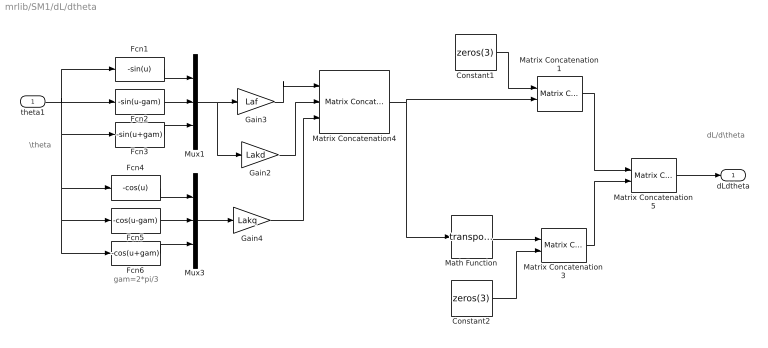
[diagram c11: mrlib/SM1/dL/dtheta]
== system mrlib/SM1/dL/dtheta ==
  note: dL/d\theta
  note: gam=2*pi/3
  note: \theta
  theta1 : Inport  OutDataType=sfix(16)  OutScaling=2^0
  Constant1 : Constant  Value=zeros(3)  VectorParams1D=off  OutDataType=sfix(16)  OutScaling=2^0
  Constant2 : Constant  Value=zeros(3)  VectorParams1D=off  OutDataType=sfix(16)  OutScaling=2^0
  Fcn1 : Fcn  Expr=-sin(u)
  Fcn2 : Fcn  Expr=-sin(u-gam)
  Fcn3 : Fcn  Expr=-sin(u+gam)
  Fcn4 : Fcn  Expr=-cos(u)
  Fcn5 : Fcn  Expr=-cos(u-gam)
  Fcn6 : Fcn  Expr=-cos(u+gam)
  Gain2 : Gain  Gain=Lakd  ParameterDataType=sfix(16)  ParameterScaling=2^0  OutDataType=sfix(16)  OutScaling=2^0
  Gain3 : Gain  Gain=Laf  ParameterDataType=sfix(16)  ParameterScaling=2^0  OutDataType=sfix(16)  OutScaling=2^0
  Gain4 : Gain  Gain=Lakq  ParameterDataType=sfix(16)  ParameterScaling=2^0  OutDataType=sfix(16)  OutScaling=2^0
  Math Function : Math  Operator=transpose
  Matrix Concatenation1 : simulink/Math Operations/Matrix Concatenation  numInports=2  catMethod=Horizontal
  Matrix Concatenation3 : simulink/Math Operations/Matrix Concatenation  numInports=2  catMethod=Horizontal
  Matrix Concatenation4 : simulink/Math Operations/Matrix Concatenation  numInports=3  catMethod=Horizontal
  Matrix Concatenation5 : simulink/Math Operations/Matrix Concatenation  numInports=2  catMethod=Vertical
  Mux1 : Mux  Inputs=3
  Mux3 : Mux  Inputs=3
  dLdtheta : Outport
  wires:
  Matrix Concatenation5/1 -> dLdtheta/1
  Matrix Concatenation4/1 -> Matrix Concatenation1/2, Math Function/1
  Mux1/1 -> Gain3/1, Gain2/1
  Matrix Concatenation1/1 -> Matrix Concatenation5/1
  Constant1/1 -> Matrix Concatenation1/1
  Fcn3/1 -> Mux1/3
  Fcn2/1 -> Mux1/2
  Fcn1/1 -> Mux1/1
  theta1/1 -> Fcn2/1, Fcn1/1, Fcn3/1, Fcn6/1, Fcn5/1, Fcn4/1
  Gain3/1 -> Matrix Concatenation4/1
  Gain2/1 -> Matrix Concatenation4/2
  Fcn5/1 -> Mux3/2
  Fcn4/1 -> Mux3/1
  Fcn6/1 -> Mux3/3
  Mux3/1 -> Gain4/1
  Gain4/1 -> Matrix Concatenation4/3
  Math Function/1 -> Matrix Concatenation3/1
  Constant2/1 -> Matrix Concatenation3/2
  Matrix Concatenation3/1 -> Matrix Concatenation5/2
